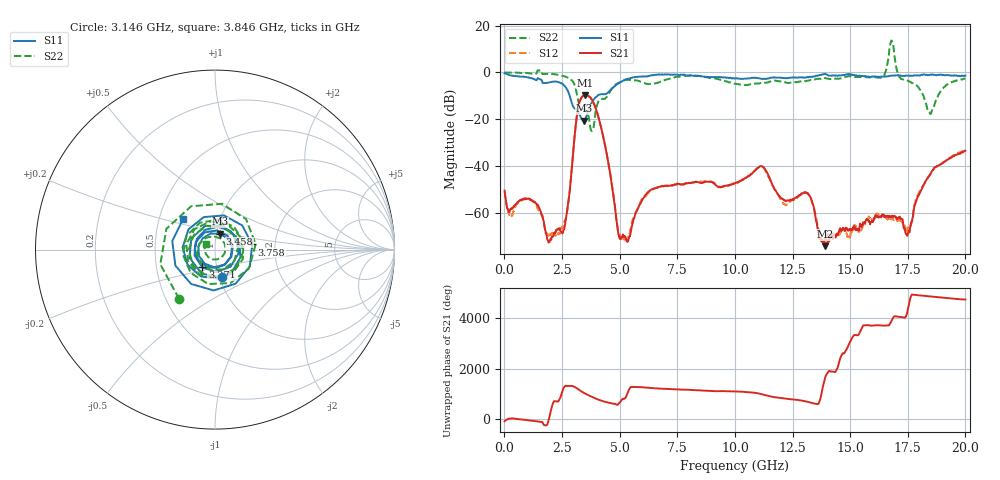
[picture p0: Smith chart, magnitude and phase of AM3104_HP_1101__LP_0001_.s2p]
!Created with skrf (http://scikit-rf.org).
# Hz S RI R 50.0
!freq ReS11 ImS11 ReS21 ImS21 ReS12 ImS12 ReS22 ImS22
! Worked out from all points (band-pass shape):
!   1601 points, 10 MHz to 20 GHz, reference 50 ohm
!   highest |S21| = -9.69 dB at 3.508 GHz (marker M1); lowest = -74.3 dB at 13.93 GHz (marker M2)
!   |S21| within 3 dB of the highest: 3.26 GHz to 3.853 GHz (593.4 MHz wide, 16.7 % of centre)
!   lowest |S11| = -20.7 dB at 3.458 GHz (marker M3), VSWR 1.20, Z = 52.1 + j9.27 ohm
!   |S11| at or under -10 dB: 2.833 GHz to 4.034 GHz (1.201 GHz wide, 35 % of centre)
!   |S22| runs from -25.0 to 13.7 dB; largest |S21 - S12| = 0.012
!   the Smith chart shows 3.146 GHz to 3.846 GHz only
!   S11 on the Smith chart (normalised r, x): 3.146 GHz: 1.03, -0.32; 3.271 GHz: 0.85, -0.17; 3.458 GHz: 1.04, +0.19; 3.758 GHz: 1.52, +0.09; 3.846 GHz: 0.66, +0.24
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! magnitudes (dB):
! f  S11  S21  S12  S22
! 10 MHz  -0.3  -50.5  -51.0  -0.1
! 2.534 GHz  -5.0  -68.2  -66.2  -1.5
! 2.771 GHz  -8.3  -55.8  -55.9  -2.4
! 3.146 GHz  -16.0  -18.6  -18.6  -9.4
! 3.271 GHz  -18.3  -12.4  -12.5  -14.5
! 3.346 GHz  -19.8  -10.8  -10.8  -15.7
! 3.458 GHz  -20.7  -9.8  -9.8  -16.0
! 3.508 GHz  -20.1  -9.7  -9.7  -16.2
! 3.758 GHz  -13.6  -11.1  -11.1  -24.8
! 3.846 GHz  -12.1  -12.5  -12.5  -24.5
! 5.02 GHz  -4.3  -71.3  -69.6  -4.1
! 6.682 GHz  -0.9  -49.0  -49.0  -4.3
! 10.01 GHz  -2.6  -47.5  -47.5  -4.9
! 11.15 GHz  -2.8  -40.1  -40.2  -4.6
! 12.14 GHz  -2.4  -54.6  -56.2  -4.1
! 13.34 GHz  -2.0  -55.1  -55.0  -3.2
! 13.93 GHz  -0.7  -74.3  -71.7  -2.5
! 16.35 GHz  -1.8  -62.0  -61.7  -2.3
! 16.68 GHz  -1.5  -62.1  -63.5  7.2
! 17.5 GHz  -1.4  -68.9  -66.8  -3.5
! 18.45 GHz  -1.0  -43.8  -44.0  -17.2
! 20 GHz  -1.4  -33.5  -33.1  -2.7
